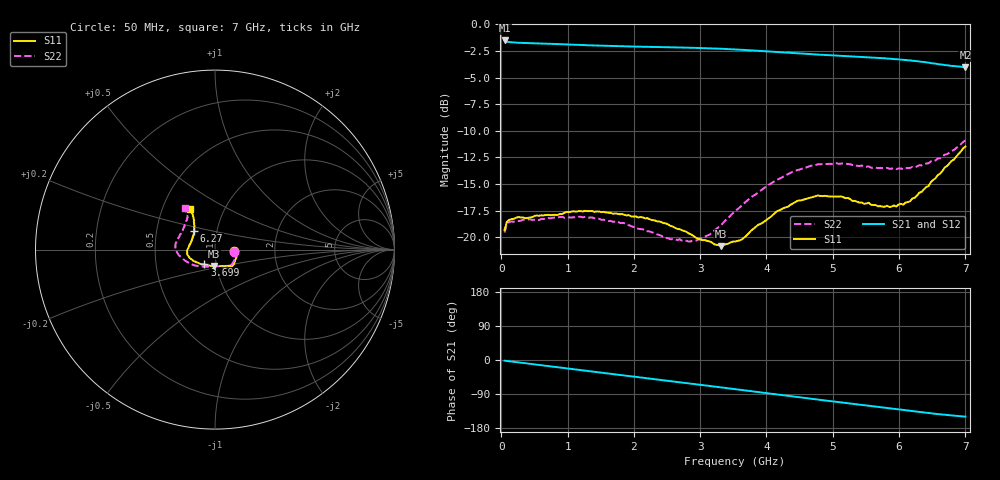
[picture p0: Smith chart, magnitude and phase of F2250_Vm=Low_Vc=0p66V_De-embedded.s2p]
! Integrated Device Technology
! Corporate Headquarters
! 6024 Silver Creek Valley Road
! San Jose, CA 95138  USA
! Phone:  1-408-284-8200
! Toll Free:  1-800-223-1366
! Webpage:  http://www.idt.com/
! Timing and RF Division
! 515 Groton Road, Suite 102
! Westford, MA 01886-6024
! Device:  F2250
! Description: Voltage Variable RF Attenuator
! Frequency:  50.0 -  6000.00 MHz
! Package:  3x3 mm Thin QFN Plastic Package: 16 pin
! Ports:  2 RF, 3 DC
!  Pin  1  = GND
!  Pin  2  = NC
!  Pin  3  = RF1  = Port 1
!  Pin  4  = NC
!  Pin  5  = GND
!  Pin  6  = GND
!  Pin  7  = GND
!  Pin  8  = GND
!  Pin  9  = NC
!  Pin 10  = RF2  = Port 2
!  Pin 11  = NC
!  Pin 12  = GND
!  Pin 13  = GND
!  Pin 14  = VCNTRL
!  Pin 15  = VDD
!  Pin 16  = VMODE
! Vcntrl:  0.660 Volts
! Vmode:  +0.000 Volts
! Vdd:  +3.30  Volts
! Current:  1.145 mA
! Data:  The device was measured on a the F2250 evaluation board which has
!  individual transmission lines to the RF pins.  Data was collected
!  using a calibrated network analyzer.  The evaluation board was
!  de-embedded using a TRL calibration technique.
!  The reference plane is the edge of the package pin.
! Misc:  SN 10
!  Action Tracker AT0258
! Date Measured:  2014-11-26
! Date:  2015-10-15  MJV
! Note:
!  Integrated Device Technology supplies this data as a sample of measured
!  data at the package pin for this product.  Your particular data for this
!  product may vary.
!  Data was taken at 25 degrees C.
!  Integrated Device Technology reserves the right to change this data at anytime.
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# GHz S dB R 50
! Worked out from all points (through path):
!   201 points, 50 MHz to 7 GHz, reference 50 ohm
!   highest |S21| = -1.51 dB at 50 MHz (marker M1); lowest = -4.0 dB at 7 GHz (marker M2)
!   group delay of S21, straight-line fit = 60 ps
!   lowest |S11| = -20.8 dB at 3.317 GHz (marker M3), VSWR 1.20, Z = 48.6 - j8.88 ohm
!   |S11| at or under -10 dB: start of sweep to end of sweep
!   |S22| runs from -20.4 to -10.9 dB; largest |S21 - S12| = 0.00065
!   S11 on the Smith chart (normalised r, x): 50 MHz: 1.24, -0.02; 3.699 GHz: 0.88, -0.15; 6.27 GHz: 0.78, +0.17; 7 GHz: 0.69, +0.34
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0.05  -19.30 -4.9  -1.51 -1.9  -1.50 -1.8  -19.54 -6.2
0.08475  -18.54 -5.2  -1.62 -2.5  -1.62 -2.5  -18.73 -6.1
0.15425  -18.29 -7.1  -1.68 -4.0  -1.68 -4.0  -18.52 -8.0
0.71025  -17.89 -25.7  -1.82 -16.2  -1.82 -16.2  -18.19 -30.9
1.2315  -17.57 -39.8  -1.94 -27.5  -1.94 -27.5  -18.12 -49.9
1.75275  -17.79 -46.5  -2.05 -38.5  -2.04 -38.5  -18.51 -60.7
2.37825  -18.52 -50.3  -2.13 -51.7  -2.13 -51.7  -19.79 -72.1
2.552  -18.93 -53.2  -2.15 -55.5  -2.15 -55.5  -20.19 -78.0
2.93425  -20.05 -66.2  -2.20 -63.9  -2.21 -63.9  -20.31 -98.2
3.14275  -20.39 -79.5  -2.25 -68.6  -2.25 -68.6  -19.76 -113.0
3.3165  -20.83 -93.9  -2.28 -72.5  -2.28 -72.5  -18.85 -124.0
3.525  -20.40 -110.9  -2.35 -77.1  -2.35 -77.1  -17.59 -135.9
3.69875  -19.83 -125.6  -2.41 -81.0  -2.41 -81.0  -16.61 -144.3
4.1505  -17.57 -150.1  -2.59 -91.0  -2.59 -91.0  -14.63 -163.7
4.7065  -16.20 -168.4  -2.81 -103.0  -2.80 -103.0  -13.27 -178.8
5.1235  -16.16 -178.5  -2.95 -112.0  -2.95 -112.0  -13.08 172.0
5.471  -16.85 170.7  -3.07 -119.3  -3.07 -119.3  -13.37 164.5
5.85325  -17.16 156.5  -3.22 -127.5  -3.22 -127.5  -13.57 154.8
6.06175  -16.94 147.4  -3.32 -132.0  -3.32 -132.0  -13.61 148.6
6.27025  -16.09 137.8  -3.46 -136.6  -3.46 -136.6  -13.34 142.0
6.61775  -14.03 125.7  -3.75 -143.2  -3.75 -143.3  -12.58 130.3
7  -11.47 121.1  -4.02 -149.5  -4.02 -149.5  -10.90 125.7
